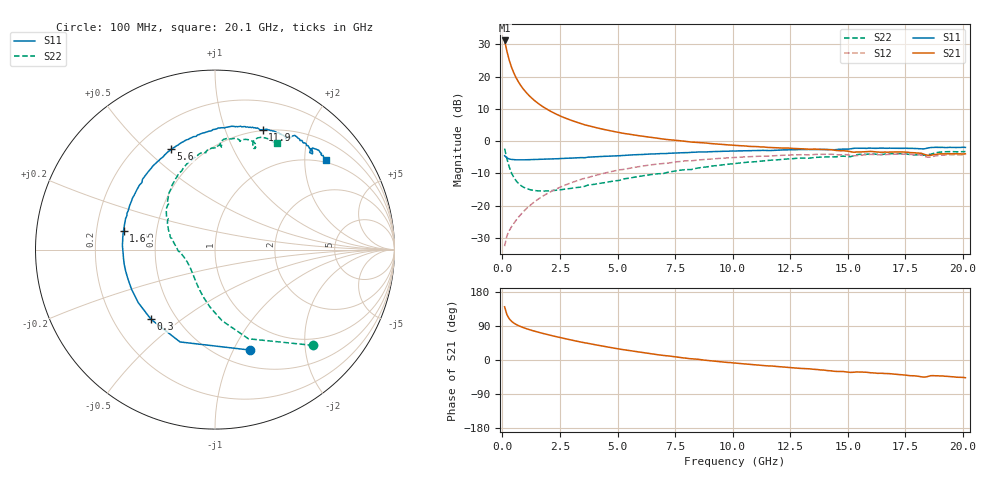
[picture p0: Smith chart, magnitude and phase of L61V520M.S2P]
!  Infineon Technologies AG
! BFR380L3 , PF131585-7, No.6, Th 09.10.01, soldered on pcb-board, measured with PP GSG850
!  Vce=1.5 V,  Ic=20.0 mA
! Common Emitter S-Parameters:  15. November 2001
#  GHz  S  MA  R  50
! f  S11  S21  S12  S22
! GHz  Mag  Ang  Mag  Ang  Mag  Ang  Mag  Ang
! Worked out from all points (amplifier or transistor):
!   201 points, 100 MHz to 20.1 GHz, reference 50 ohm
!   highest |S21| = 31.2 dB at 100 MHz (marker M1)
!   |S21| within 3 dB of that: start of sweep to 189.7 MHz
!   unconditionally stable (mu >= 1): 1.346 GHz to 4.634 GHz
!   at 3.4 GHz: K = 1.02, MAG = 7.8 dB, |S12| = -11.9 dB
!   at 10.1 GHz: K = 0.97, MSG = 1.9 dB, |S12| = -5.1 dB
!   at 20.1 GHz: K = 0.99, MSG = 0.1 dB, |S12| = -4.2 dB
!   S11 on the Smith chart (normalised r, x): 100 MHz: 0.67, -1.16; 300 MHz: 0.36, -0.39; 1.6 GHz: 0.32, +0.09; 5.6 GHz: 0.34, +0.60; 11.9 GHz: 0.49, +1.36; 20.1 GHz: 0.92, +2.54
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0.1  0.5921 -70.9  36.17 140.4  0.02355 62.5  0.7642 -44.3
0.2  0.5502 -110.8  24.61 119.6  0.03397 53.9  0.5306 -69.5
0.3  0.5272 -132.6  17.93 108.9  0.04089 53.2  0.3976 -84.4
0.4  0.5198 -145.4  13.94 102.2  0.0471 54.2  0.3207 -95.1
0.5  0.5149 -154.3  11.34 97.4  0.05312 56.1  0.2735 -103.5
0.6  0.512 -160.9  9.551 93.8  0.05962 58.1  0.2425 -110.4
0.7  0.5119 -166.2  8.257 90.7  0.06609 59.4  0.2209 -116.4
0.8  0.5123 -170.3  7.258 88.1  0.07276 60.6  0.2057 -121.6
0.9  0.512 -173.9  6.479 85.7  0.07969 61.6  0.1947 -126.2
1.1  0.5143 180.0  5.344 81.6  0.09355 62.8  0.1814 -134.0
1.3  0.5166 174.9  4.549 77.8  0.1076 63.3  0.1734 -140.4
1.6  0.5199 168.3  3.728 72.7  0.129 63.2  0.169 -148.0
2  0.5273 160.9  3.022 66.5  0.1573 62.0  0.1693 -156.0
2.4  0.5329 154.0  2.554 60.7  0.1855 60.3  0.1736 -162.8
3.5  0.5525 138.0  1.823 46.3  0.2606 53.8  0.195 -176.4
5.6  0.6097 113.6  1.263 24.2  0.3836 39.5  0.2704 160.2
6.8  0.6374 101.8  1.095 13.4  0.4442 30.9  0.312 147.4
10.1  0.7001 77.6  0.8569 -8.0  0.5569 9.6  0.4489 119.7
11.9  0.7192 68.3  0.7909 -16.9  0.5957 -0.9  0.5112 105.5
13.5  0.7395 60.5  0.7504 -24.5  0.6169 -10.5  0.5527 94.7
16.8  0.7767 48.2  0.6752 -36.0  0.622 -26.0  0.6348 75.2
20.1  0.7975 38.9  0.6347 -46.8  0.6158 -39.3  0.6881 59.8
